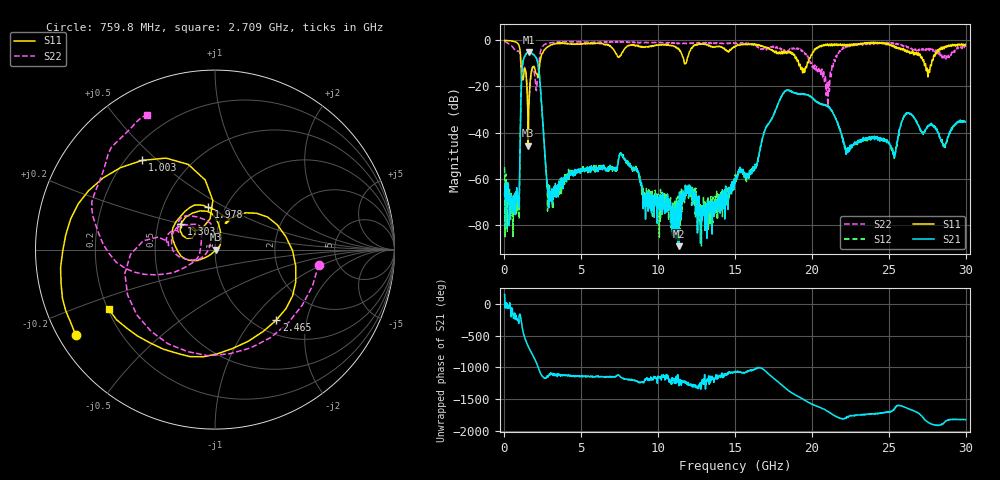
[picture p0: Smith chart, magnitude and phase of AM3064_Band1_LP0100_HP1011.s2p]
# Hz S DB R 50.0
!freq dBS11 angS11 dBS21 angS21 dBS12 angS12 dBS22 angS22
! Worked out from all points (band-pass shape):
!   1600 points, 10 MHz to 29.98 GHz, reference 50 ohm
!   highest |S21| = -5.13 dB at 1.584 GHz (marker M1); lowest = -89.3 dB at 11.35 GHz (marker M2)
!   |S21| within 3 dB of the highest: 1.245 GHz to 2.1 GHz (855.3 MHz wide, 51.1 % of centre)
!   lowest |S11| = -45.7 dB at 1.547 GHz (marker M3), VSWR 1.01, Z = 50.5 - j0.0546 ohm
!   |S11| at or under -10 dB: 1.071 GHz to 2.301 GHz (1.23 GHz wide, 73 % of centre); 19.13 GHz to 19.69 GHz (553.6 MHz wide, 2.85 % of centre); 27.3 GHz to 27.78 GHz (480.8 MHz wide, 1.75 % of centre)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
!   |S22| runs from -29.4 to -0.4 dB; largest |S21 - S12| = 0.0077
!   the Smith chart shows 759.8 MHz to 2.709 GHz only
!   S11 on the Smith chart (normalised r, x): 759.8 MHz: 0.05, -0.28; 1.003 GHz: 0.27, +0.45; 1.303 GHz: 0.66, +0.20; 1.978 GHz: 0.83, +0.42; 2.465 GHz: 1.24, -1.34; 2.709 GHz: 0.20, -0.25
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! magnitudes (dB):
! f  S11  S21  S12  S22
! 10 MHz  -0.1  -66.7  -55.1  -0.4
! 759.8 MHz  -0.8  -65.5  -70.4  -4.7
! 1.003 GHz  -3.9  -50.8  -50.2  -5.7
! 1.303 GHz  -12.5  -7.1  -7.1  -11.8
! 1.547 GHz  -45.7  -5.2  -5.1  -28.9
! 1.584 GHz  -29.2  -5.1  -5.1  -28.4
! 1.978 GHz  -12.5  -6.7  -6.7  -15.8
! 2.465 GHz  -5.7  -32.7  -32.7  -2.7
! 2.709 GHz  -3.4  -57.4  -57.1  -1.5
! 3.028 GHz  -2.0  -66.3  -67.8  -1.0
! 5.015 GHz  -1.5  -56.7  -56.8  -0.6
! 7.601 GHz  -6.1  -49.1  -48.7  -0.7
! 10 GHz  -2.0  -72.9  -72.0  -1.0
! 11.35 GHz  -3.9  -89.3  -69.7  -1.3
! 15 GHz  -2.8  -61.3  -58.6  -1.4
! 18.21 GHz  -5.6  -22.4  -22.3  -4.3
! 19.99 GHz  -6.3  -24.9  -24.8  -10.8
! 21.02 GHz  -1.7  -28.6  -28.7  -26.1
! 22.28 GHz  -2.5  -47.4  -46.9  -2.2
! 25 GHz  -1.5  -44.1  -44.3  -1.2
! 27.56 GHz  -15.2  -37.3  -37.3  -3.7
! 29.98 GHz  -1.7  -35.3  -35.0  -2.9
